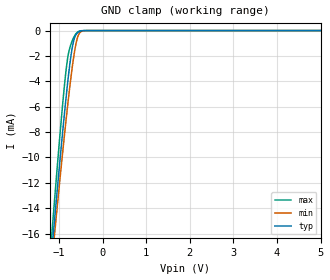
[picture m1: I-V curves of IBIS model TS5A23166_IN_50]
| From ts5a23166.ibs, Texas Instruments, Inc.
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[Model]   TS5A23166_IN_50
Model_type  Input
Vinl=0.8
Vinh=2.4
| variable   typ   min   max
C_comp   1.56pF   1.23pF   2.07pF
[Temperature Range]   40   100   -40
| Ambient temperature   25   85   -40
[Voltage range]   5   4.5   5.5
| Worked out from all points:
|   GND clamp passes 1 mA (typ) near -0.68 V on its own axis
[GND Clamp]
| TS5A23166_IN_50
|   Voltage   I(typ)   I(min)   I(max)
-5V       -184.3mA   -172.6mA   -197.7mA
-1.175V   -17.77mA   -18.67mA   -16.5mA
-1.14V    -16.4mA    -17.41mA   -14.99mA
-1.105V   -15.04mA   -16.16mA   -13.49mA
-1.075V   -13.89mA   -15.09mA   -12.22mA
-920mV    -8.126mA   -9.736mA   -5.957mA
-815mV    -4.545mA   -6.325mA   -2.498mA
-760mV    -2.885mA   -4.658mA   -1.463mA
-685mV    -1.138mA   -2.611mA   -710.2uA
-610mV    -320.4uA   -1.034mA   -241.2uA
-545mV    -94.2uA    -287.3uA   -57.32uA
5V        94.64pA    195.7pA    60.23pA
